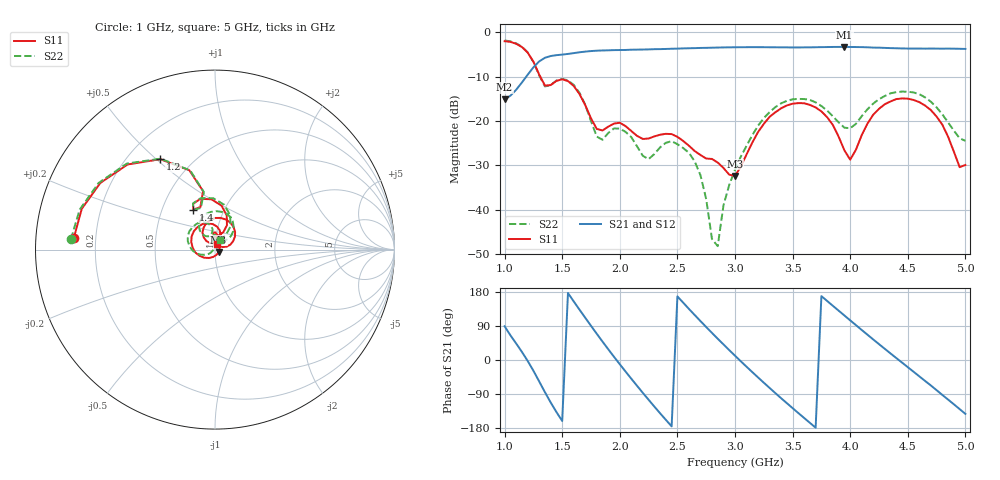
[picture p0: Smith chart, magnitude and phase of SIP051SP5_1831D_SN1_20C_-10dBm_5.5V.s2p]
# GHz  S  dB  R  50
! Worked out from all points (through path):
!   81 points, 1 GHz to 5 GHz, reference 50 ohm
!   highest |S21| = -3.33 dB at 3.95 GHz (marker M1); lowest = -15.1 dB at 1 GHz (marker M2)
!   lowest |S11| = -32.4 dB at 3 GHz (marker M3), VSWR 1.05, Z = 52 - j1.43 ohm
!   |S11| at or under -10 dB: 1.309 GHz to end of sweep
!   |S22| runs from -48.2 to -1.9 dB; largest |S21 - S12| = 0.0023
!   S11 on the Smith chart (normalised r, x): 1 GHz: 0.12, +0.04; 1.2 GHz: 0.33, +0.52; 1.4 GHz: 0.72, +0.34; 5 GHz: 1.02, +0.06
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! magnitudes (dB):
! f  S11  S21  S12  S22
! 1 GHz  -2.1  -15.1  -15.1  -1.9
! 1.2 GHz  -4.6  -9.6  -9.6  -4.6
! 1.4 GHz  -11.9  -5.4  -5.4  -12.0
! 1.55 GHz  -11.0  -4.9  -4.9  -10.9
! 1.7 GHz  -16.4  -4.4  -4.4  -16.4
! 1.8 GHz  -21.8  -4.2  -4.2  -23.5
! 2 GHz  -20.4  -4.0  -4.0  -21.7
! 2.25 GHz  -23.9  -3.9  -3.9  -28.6
! 2.35 GHz  -23.1  -3.8  -3.8  -25.9
! 2.65 GHz  -26.8  -3.6  -3.6  -29.1
! 2.75 GHz  -28.4  -3.5  -3.5  -37.6
! 2.8 GHz  -28.5  -3.5  -3.5  -46.5
! 2.85 GHz  -29.3  -3.5  -3.5  -48.2
! 2.9 GHz  -30.6  -3.5  -3.5  -39.0
! 3 GHz  -32.4  -3.4  -3.4  -31.0
! 3.3 GHz  -19.1  -3.4  -3.4  -18.0
! 3.7 GHz  -17.0  -3.4  -3.4  -15.8
! 3.95 GHz  -26.6  -3.3  -3.3  -21.5
! 4 GHz  -28.7  -3.4  -3.4  -21.6
! 4.35 GHz  -15.6  -3.6  -3.6  -13.8
! 4.7 GHz  -17.5  -3.7  -3.7  -15.7
! 5 GHz  -29.9  -3.8  -3.8  -24.5
